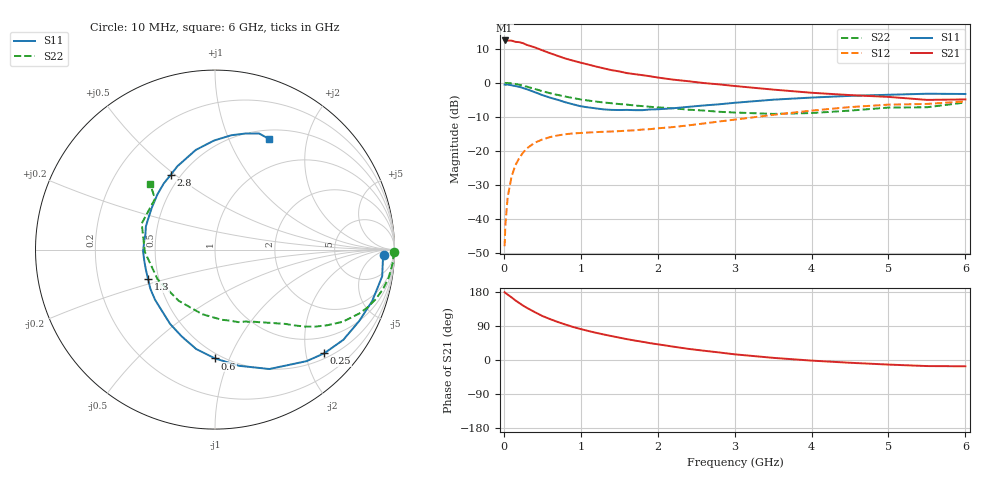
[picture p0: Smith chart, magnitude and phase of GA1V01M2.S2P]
! Infineon Technologies  Discrete & RF Semiconductors
! BF775
! Si NPN RF Bipolar Junction Transistor in SOT23
! VCE = 1 V  IC = 1.2 mA
! Common Emitter S-Parameters:  May  1996
# GHz  S  MA  R  50
!  f  S11  S21  S12  S22
! GHz  MAG  ANG  MAG  ANG  MAG  ANG  MAG  ANG
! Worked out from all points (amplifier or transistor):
!   36 points, 10 MHz to 6 GHz, reference 50 ohm
!   highest |S21| = 12.4 dB at 10 MHz (marker M1)
!   |S21| within 3 dB of that: start of sweep to 513.1 MHz
!   unconditionally stable (mu >= 1): 1.273 GHz to end of sweep
!   at 250 MHz: K = 0.23, MSG = 16.1 dB, |S12| = -20.5 dB
!   at 1.4 GHz: K = 1.08, MAG = 7.3 dB, |S12| = -14.3 dB
!   at 6 GHz: K = 1.08, MAG = -1.4 dB, |S12| = -5.5 dB
!   S11 on the Smith chart (normalised r, x): 10 MHz: 27, -15; 250 MHz: 0.61, -2.37; 600 MHz: 0.46, -0.89; 1.3 GHz: 0.44, -0.17; 2.8 GHz: 0.44, +0.48; 6 GHz: 0.61, +1.42
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0.01  0.9443 -1.8  4.191 178.9  0.004 87.5  0.9992 -0.8
0.02  0.9372 -3.5  4.087 176.9  0.0082 86.7  0.9956 -1.8
0.05  0.9433 -9.1  4.18 172.6  0.0211 83.0  0.9923 -4.5
0.1  0.9213 -18.2  4.171 165.3  0.0419 78.9  0.9807 -9.1
0.15  0.8965 -26.4  3.998 157.4  0.0614 73.3  0.9618 -13.2
0.2  0.874 -35.1  3.957 150.4  0.0788 68.7  0.9373 -17.1
0.25  0.8393 -43.5  3.818 143.6  0.0946 63.5  0.9068 -21.0
0.3  0.8043 -50.6  3.602 137.6  0.1093 59.8  0.8781 -24.0
0.4  0.7311 -65.5  3.324 126.6  0.1318 52.3  0.817 -29.5
0.5  0.6612 -78.3  3.005 116.2  0.1473 46.3  0.7538 -34.0
0.6  0.6063 -90.0  2.726 108.0  0.1599 41.7  0.7048 -37.5
0.8  0.5184 -110.9  2.275 93.6  0.1759 35.1  0.6288 -42.5
0.9  0.4839 -121.1  2.118 87.2  0.1809 33.1  0.5978 -44.6
1.1  0.4356 -140.0  1.854 76.5  0.1867 30.3  0.5491 -48.6
1.3  0.4075 -156.3  1.63 67.3  0.1916 28.9  0.5145 -52.3
1.7  0.3974 173.1  1.343 51.4  0.2009 29.4  0.465 -60.1
2.2  0.4234 145.9  1.115 35.3  0.2241 32.0  0.4241 -72.3
2.8  0.4845 120.5  0.949 19.9  0.2709 33.6  0.3757 -92.5
3.5  0.5656 100.9  0.796 5.7  0.3389 30.1  0.3497 -125.3
4.5  0.6436 81.9  0.661 -7.3  0.4407 18.8  0.3911 -178.1
5.5  0.692 69.2  0.562 -16.0  0.4903 4.1  0.4382 139.7
6  0.6862 64.0  0.571 -16.6  0.5338 0.0  0.5153 134.6
